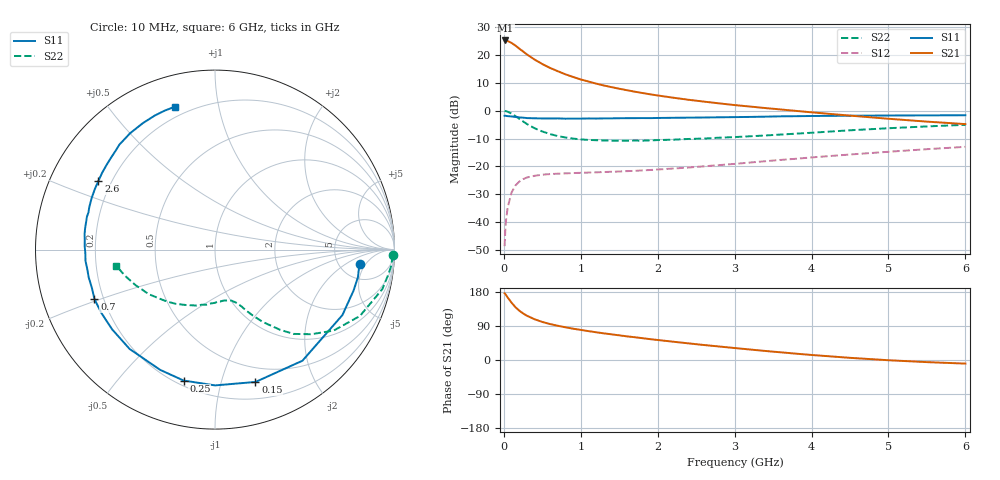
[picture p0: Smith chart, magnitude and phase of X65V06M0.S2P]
! SIEMENS Small Signal Semiconductors
! BFP193W
! Si NPN RF Bipolar Junction Transistor in SOT343
! VCE = 5 V  IC = 6 mA
! Common Emitter S-Parameters:  April 1994
# GHz  S  MA  R  50
!  f  S11  S21  S12  S22
! GHz  MAG  ANG  MAG  ANG  MAG  ANG  MAG  ANG
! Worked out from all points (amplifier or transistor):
!   40 points, 10 MHz to 6 GHz, reference 50 ohm
!   highest |S21| = 25.2 dB at 20 MHz (marker M1)
!   |S21| within 3 dB of that: start of sweep to 204.6 MHz
!   unconditionally stable (mu >= 1): 1.623 GHz to 4.42 GHz
!   at 200 MHz: K = 0.16, MSG = 23.9 dB, |S12| = -25.5 dB
!   at 1.5 GHz: K = 0.95, MSG = 14.9 dB, |S12| = -21.8 dB
!   at 6 GHz: K = 0.92, MSG = 4.1 dB, |S12| = -13.0 dB
!   lowest NFmin = 1.20 dB at 450 MHz
!   S11 on the Smith chart (normalised r, x): 10 MHz: 7.86, -3.53; 150 MHz: 0.35, -1.29; 250 MHz: 0.23, -0.76; 700 MHz: 0.16, -0.19; 2.6 GHz: 0.15, +0.27; 6 GHz: 0.15, +0.75
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0.01  0.8089 -5.5  18.16 176.1  0.0037 85.1  0.9912 -1.9
0.02  0.8111 -11.0  18.2 173.8  0.0076 82.8  0.9851 -5.5
0.05  0.7981 -27.2  17.76 164.9  0.0183 76.0  0.9578 -13.3
0.1  0.7878 -51.8  16.42 151.4  0.0339 64.6  0.8882 -24.6
0.15  0.7712 -73.0  14.76 139.5  0.0453 54.8  0.8004 -34.3
0.2  0.7566 -90.0  13.03 130.3  0.0533 47.6  0.7144 -41.3
0.25  0.7502 -103.5  11.56 123.0  0.0591 41.9  0.6423 -47.0
0.3  0.7365 -114.5  10.22 116.8  0.0632 37.6  0.5761 -50.9
0.4  0.7299 -130.7  8.261 107.5  0.0678 31.7  0.4841 -56.5
0.5  0.7252 -142.2  6.871 100.4  0.071 28.4  0.4231 -60.2
0.6  0.7248 -150.7  5.852 94.9  0.0728 26.2  0.3806 -63.0
0.7  0.7262 -157.6  5.115 90.4  0.0739 25.1  0.3504 -64.9
0.9  0.7205 -167.5  4.029 82.6  0.0759 24.5  0.3156 -68.7
1.1  0.7244 -175.1  3.334 76.2  0.0775 24.9  0.2982 -72.2
1.3  0.7263 178.5  2.832 70.3  0.0792 26.3  0.2915 -76.1
1.6  0.7335 170.6  2.33 62.4  0.0822 28.9  0.2888 -81.8
2.2  0.7449 157.3  1.71 48.3  0.0915 34.6  0.3013 -94.7
2.6  0.7539 149.5  1.455 39.6  0.1002 38.2  0.316 -103.6
3.2  0.7724 138.9  1.186 27.7  0.1172 41.3  0.3471 -117.0
4.5  0.8112 119.7  0.815 5.7  0.1634 41.4  0.4445 -146.0
5.5  0.8232 110.1  0.636 -5.6  0.2035 37.6  0.5219 -163.7
6  0.8273 105.6  0.574 -9.5  0.2245 35.4  0.5572 -170.7
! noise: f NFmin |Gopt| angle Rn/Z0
0.45  1.2  0.25  114  0.13
0.9  1.25  0.37  150  0.12
1.8  2  0.55  -158  0.12
